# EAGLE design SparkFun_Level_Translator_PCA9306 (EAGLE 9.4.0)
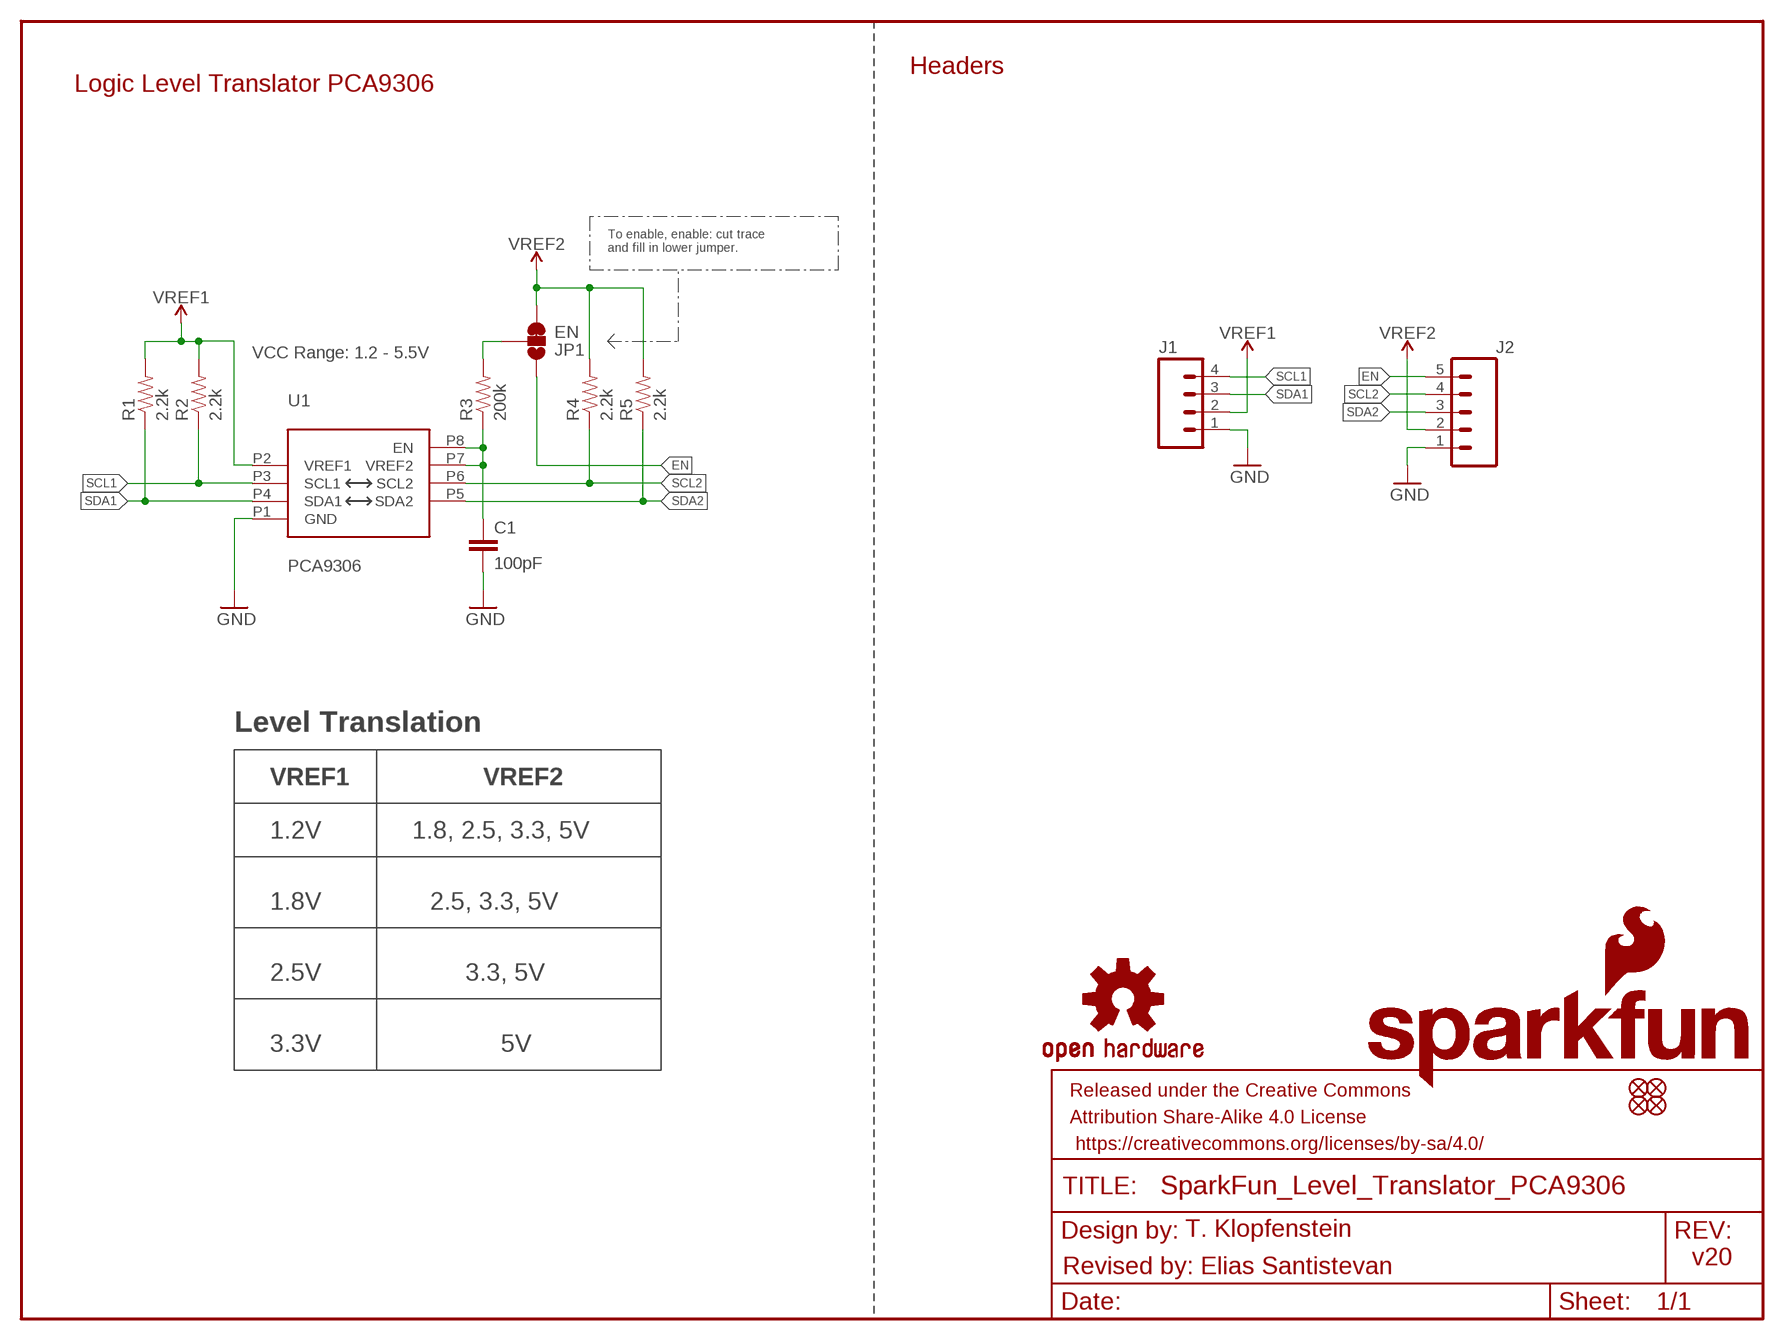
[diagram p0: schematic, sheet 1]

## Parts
C1  100pF  100PF-0603-50V-5%  [0603]
FD1  FIDUCIALUFIDUCIAL  [FIDUCIAL-MICRO]
FD2  FIDUCIALUFIDUCIAL  [FIDUCIAL-MICRO]
FD3  FIDUCIALUFIDUCIAL  [FIDUCIAL-MICRO]
FD4  FIDUCIALUFIDUCIAL  [FIDUCIAL-MICRO]
FRAME1  FRAME-LETTER  [CREATIVE_COMMONS]
J1  CONN_041X04_NO_SILK  [1X04_NO_SILK]
J2  CONN_05NO_SILK  [1X05_NO_SILK]
JP1  EN  JUMPER-SMT_3_1-NC_TRACE_SILK  [SMT-JUMPER_3_1-NC_TRACE_SILK]
LOGO1  OSHW-LOGOMINI  [OSHW-LOGO-MINI]
LOGO2  SFE_LOGO_NAME.1_INCH  [SFE_LOGO_NAME_.1]
LOGO3  SFE_LOGO_FLAME.1_INCH  [SFE_LOGO_FLAME_.1]
R1  2.2k  2.2KOHM-0603-1/10W-1%  [0603]
R2  2.2k  2.2KOHM-0603-1/10W-1%  [0603]
R3  200k  200KOHM-0603-1/10W-1%  [0603]
R4  2.2k  2.2KOHM-0603-1/10W-1%  [0603]
R5  2.2k  2.2KOHM-0603-1/10W-1%  [0603]
U1  PCA9306  PCA9306VSSOP_8PIN  [VSSOP_8PIN]

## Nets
EN: J2.5 JP1.1
GND: C1.2 J1.1 J2.1 U1.P1(GND)
JUMPER_IN: JP1.2 R3.2
SCL1: J1.4 R2.1 U1.P3(SCL1)
SCL2: J2.4 R4.1 U1.P6(SCL2)
SDA1: J1.3 R1.1 U1.P4(SDA1)
SDA2: J2.3 R5.1 U1.P5(SDA2)
VREF1: J1.2 R1.2 R2.2 U1.P2(VREF1)
VREF2: J2.2 JP1.3 R4.2 R5.2
VREF2_IN: C1.1 R3.1 U1.P7(VREF2) U1.P8(EN)

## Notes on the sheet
- Headers
- Logic Level Translator PCA9306
- To enable, enable: cut trace
  and fill in lower jumper.
- VCC Range: 1.2 - 5.5V
- Level Translation
- VREF1 | VREF2
- 1.2V | 1.8, 2.5, 3.3, 5V
- 1.8V | 2.5, 3.3, 5V
- 2.5V | 3.3, 5V
- 3.3V | 5V
- T. Klopfenstein
- v20
- Revised by: Elias Santistevan

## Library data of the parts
C1 = SparkFun-Capacitors:100PF: 100pF/0.1nF ceramic capacitors; PROD_ID: CAP-07883
FD1-FD4 = SparkFun-Aesthetics:FIDUCIAL: Fiducial Alignment Points
FRAME1 = SparkFun-Aesthetics:FRAME-LETTER: Schematic Frame - Letter
J1 = SparkFun-Connectors:CONN_04: Multi connection point. Often used as Generic Header-pin footprint for 0.1 inch spaced/style header connections On any of the 0.1 inch spaced packages, you can populate with these: Break Away Headers - Straight (PRT-00116) Break Away Male Headers - Right Angle (PRT-00553) Female Headers (PRT-00115)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; PROD_ID: CONN-09696
J2 = SparkFun-Connectors:CONN_05: Multi connection point. Often used as Generic Header-pin footprint for 0.1 inch spaced/style header connections On any of the 0.1 inch spaced packages, you can populate with these: Break Away Headers - Straight (PRT-00116) Break Away Male Headers - Right Angle (PRT-00553) Female Headers (PRT-00115)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
JP1 = SparkFun-Jumpers:JUMPER-SMT_3_1-NC_TRACE: Normally closed trace jumper (1 of 2 connections) This jumper has a trace between two pads so it's normally closed (NC). The other connection is normally open (NO). Use a razor knife to open the connection. For best results follow the IPC guidelines for cutting traces: Cutout at least 0.063 mm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
LOGO1 = SparkFun-Aesthetics:OSHW-LOGO: Open-Source Hardware (OSHW) Logo
LOGO2 = SparkFun-Aesthetics:SFE_LOGO_NAME: SparkFun Font Logo
LOGO3 = SparkFun-Aesthetics:SFE_LOGO_FLAME: SparkFun Flame Logo
R1 R2 R4 R5 = SparkFun-Resistors:2.2KOHM: 2.2kΩ resistor; PROD_ID: RES-08272
R3 = SparkFun-Resistors:200KOHM: 200kΩ resistor; PROD_ID: RES-09385
U1 = SparkFun-IC-Comms:PCA9306: Bidirectional I2C level shifter Not compatible with all available part number pinout schemes- DOUBLE CHECK!!! Variants PCA9306DC and PSOP-8 are EOL. If your part has VREF as pin 1 then this is your variant. VSSOP_8PIN is not EOL. Datasheet SparkFun Products SparkFun Inventor's Kit for RedBot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; PROD_ID: IC-14450

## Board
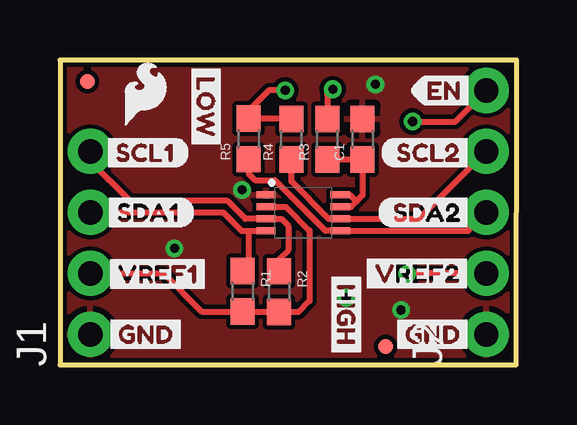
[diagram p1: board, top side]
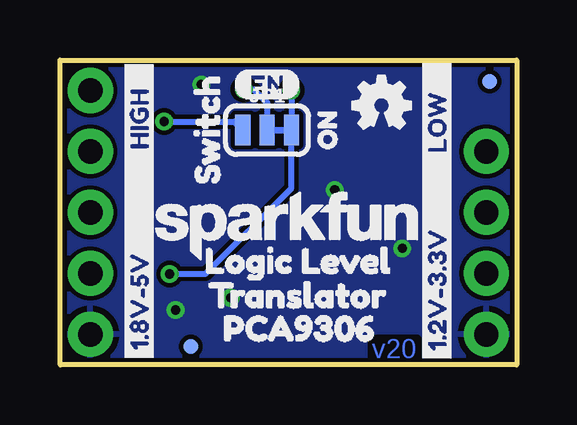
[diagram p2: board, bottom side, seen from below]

Size 19.05 x 12.7 mm. Coordinates in mm from the lower left corner, seen from the top.
Outline: 0,0 19.03,0 19.05,12.7 0,12.7 0,0
Copper layers (1*16): Top 0.035mm / dielectric 1.5mm / Bottom 0.035mm
Design rules "SparkFun-2-layer-TIGHT": minimum track width 7mil, minimum drill 15mil, track to track 7mil, track to pad 7mil, pad to pad 7mil, via to via 7mil, smd to smd 7mil, copper to edge 7mil, drill to drill 7mil, minimum pad ring 7mil, minimum via ring 7mil, stop-mask expansion 4mil, vias tented up to drill 25mil, thermal gap 10mil

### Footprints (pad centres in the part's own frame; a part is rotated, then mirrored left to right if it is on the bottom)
0603 = smd 1.1 x 1: 1 -0.85,0; 2 0.85,0
FIDUCIAL-MICRO = smd 0.635 x 0.635: 1 0,0
1X04_NO_SILK = drill 1.016 pad 1.88: 1 0,0; 2 2.54,0; 3 5.08,0; 4 7.62,0
1X05_NO_SILK = drill 1.016 pad 1.88: 1 0,0; 2 2.54,0; 3 5.08,0; 4 7.62,0; 5 10.16,0
SMT-JUMPER_3_1-NC_TRACE_SILK = smd 0.635 x 1.27: 1 -1.016,0; 2 0,0; 3 1.016,0
VSSOP_8PIN = smd 0.8 x 0.3: P1 -1.57,0.734; P2 -1.57,0.234; P3 -1.57,-0.266; P4 -1.57,-0.766; P5 1.53,-0.766; P6 1.53,-0.266; P7 1.53,0.234; P8 1.53,0.734

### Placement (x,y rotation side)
C1  12.62,9.4 90 top
FD1  1.14,11.81 90 bottom
FD2  13.59,0.76 90 top
FD3  1.14,11.81 90 top
FD4  13.59,0.76 90 bottom
FRAME1  not placed on the board
J1  1.27,1.27 90 top
J2  17.78,1.27 90 top
JP1  10.41,9.78 0 bottom
LOGO1  5.64,10.82 0 bottom
LOGO2  9.58,5.79 0 bottom
LOGO3  3.56,11.3 0 top
R1  7.62,3.06 270 top
R2  9.14,3.05 270 top
R3  11.15,9.4 90 top
R4  9.65,9.4 90 top
R5  7.87,9.41 90 top
U1  10.16,6.35 0 top
U$1  [SWITCH1]  12.9,6.6 90 bottom
U$2  [VREF13]  1.7,3.78 0 top
U$3  [SCL11]  1.63,8.84 0 top
U$4  [SDA10]  1.7,6.35 0 top
U$5  [GND2]  1.75,1.27 0 top
U$6  [VREF20]  12.45,3.81 0 top
U$7  [SCL20]  13.36,8.84 0 top
U$8  [SDA21]  13.21,6.35 0 top
U$9  [EN0]  14.61,11.43 0 top
U$10  [EN1]  11.81,11.68 0 bottom
U$11  [GND2]  13.72,1.27 0 top
U$12  [LOGIC_LEVEL0]  13.92,4.34 0 bottom
U$13  [TRANSLATOR1]  13.77,2.9 0 bottom
U$14  [PCA93062]  13.16,1.52 0 bottom
U$15  [ON2]  7.9,8.18 90 bottom
U$17  [HIGH0]  15.75,8.28 90 bottom
U$18  [LOW1]  3.33,8.15 90 bottom
U$19  [HIGH0]  11.94,4.06 270 top
U$20  [LOW1]  6.1,12.7 270 top
U$21  [1#2V#3#3V0]  3.33,-0.13 90 bottom
U$22  [1#8V#5V1]  15.75,-0.1 90 bottom

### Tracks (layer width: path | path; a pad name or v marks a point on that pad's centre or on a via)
EN  (via drill 0.38)
  Top 0.254: v14.71,10.13 16.48,10.13 J2.5
  Bottom 0.254: JP1.1 11.79,10.13 v14.71,10.13
GND  (via drill 0.38)
  other vias: 7.59,7.29 4.78,4.85 11.94,2.79 13.16,11.68 14.22,2.29
  pour Bottom: 0,12.7 19.05,12.7 19.05,0 0,0
  pour Top: 0,12.7 19.05,12.7 19.05,0 0,0
JUMPER_IN  (via drill 0.38)
  Top 0.254: v11.38,11.48 11.15,11.25 R3.2
  Bottom 0.254: v11.38,11.48 10.97,11.48 10.41,10.92 JP1.2
SCL1
  Top 0.254: R2.1 9.14,4.39 9.53,4.78 9.53,5.79 9.23,6.08 U1.P3 7.73,6.08 6.99,6.83 2.92,6.83 1.27,8.48 J1.4
SCL2
  Top 0.254: R4.1 9.65,7.64 11.21,6.08 U1.P6 14.97,6.08 J2.4
SDA1
  Top 0.254: J1.3 6.81,6.35 7.57,5.58 7.87,5.58 | 7.87,5.58 U1.P4 | 7.87,5.58 7.87,4.17 R1.1
SDA2
  Top 0.254: J2.3 17.01,5.58 U1.P5 11.07,5.58 8.97,7.69 8.14,7.69 7.87,7.96 R5.1
VREF1
  Top 0.254: J1.2 4.32,3.81 5.91,2.21 R1.2 9.13,2.21 R2.2 9.95,2.2 10.41,2.67 10.41,5.59 9.42,6.58 U1.P2
VREF2  (via drill 0.38)
  Top 0.254: R4.2 7.89,10.25 R5.2 7.87,10.59 8.71,11.43 v9.4,11.43 | J2.2 14.48,3.81 v14.48,3.79
  Bottom 0.254: v9.4,11.43 JP1.3 9.4,7.37 12.98,3.79 v14.48,3.79
VREF2_IN
  Top 0.254: R3.1 C1.1 12.62,7.06 12.37,6.81 | 12.37,6.81 12.15,6.58 U1.P7 | U1.P8 12.09,7.08 12.37,6.81

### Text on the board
Bottom: v20
tValues: T. Klopfenstein
Measures: Units in Inches
tDocu: Toni Klopfenstein | Revised by: Elias Santistevan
